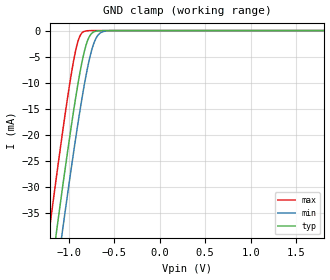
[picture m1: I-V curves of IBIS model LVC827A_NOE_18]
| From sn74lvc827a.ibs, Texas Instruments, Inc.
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[Model]   LVC827A_NOE_18
Model_type  Input
Vinl = 0.5775
Vinh = 1.2675
| variable   typ   min   max
C_comp   4.05pF   3.23pF   4.78pF
[Temperature Range]   40   100   -40
| Ambient temperature   25   85   -40
[Voltage range]   1.8   1.65   1.95
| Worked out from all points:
|   GND clamp passes 1 mA (typ) near -0.77 V on its own axis
[GND Clamp]
| LVC827A_NOE_18
|   Voltage   I(typ)   I(min)   I(max)
-5V       -584.4mA   -591.4mA   -575.6mA
-1.21V    -48.98mA   -57.27mA   -38.33mA
-1.135V   -39.11mA   -47.4mA    -28.45mA
-1.075V   -31.38mA   -39.64mA   -20.77mA
-1.06V    -29.47mA   -37.73mA   -18.9mA
-960mV    -17.27mA   -25.29mA   -7.384mA
-885mV    -9.107mA   -16.56mA   -1.487mA
-830mV    -4.285mA   -10.76mA   -171.7uA
-780mV    -1.473mA   -6.233mA   -17.16uA
-715mV    -205.6uA   -2.13mA    -809.3nA
-650mV    -22.03uA   -444.3uA   -37.97nA
1.8V      3.326pA    6.145pA    3.026pA
